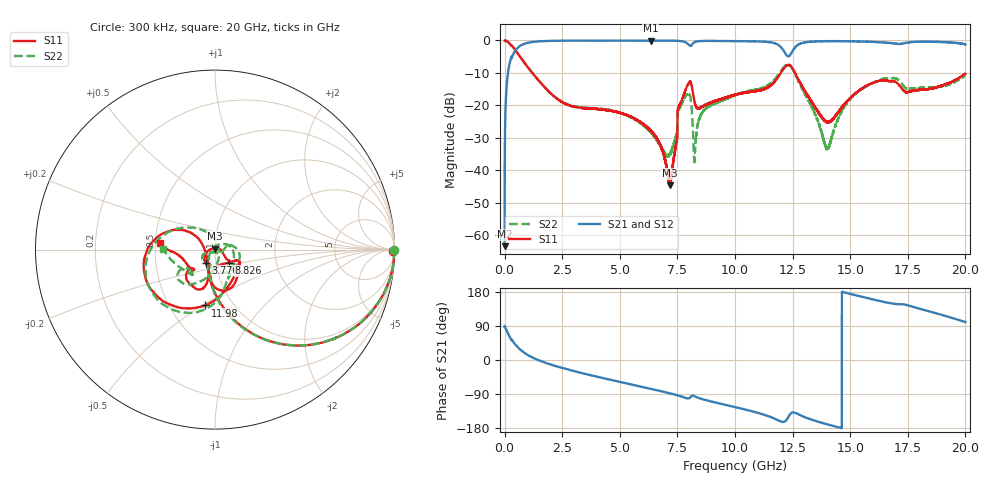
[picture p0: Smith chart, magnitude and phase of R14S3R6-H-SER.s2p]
!{R14S3R6}
!Johanson Technology Inc.
!www.johansontechnology.com
!Test Board Conditions:
!Substrate Type  RO4350B
!Substrate Thickness  20 mil
!Substrate Dk  3.66
!TL Type: GCPW
!TL Trace Width  36 mil
!TL Gap  12 mil
!Electrode orientation  Horizontal
!DUT TOPOLOGY	SERIES
!Mounting Pad LxW  26x36 mil
! Created Wed Nov 25 17:33:21 2020
! 2 Port Network Data from SP1.SP block
! freq  magS11  angS11  magS21  angS21  magS12  angS12  magS22  angS22
# khz S ma R 50
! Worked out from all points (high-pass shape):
!   20001 points, 300 kHz to 20 GHz, reference 50 ohm
!   highest |S21| = -0.05 dB at 6.349 GHz (marker M1); lowest = -63.4 dB at 300 kHz (marker M2)
!   |S21| within 3 dB of the highest: 471 MHz to 12.1 GHz (11.63 GHz wide, 185 % of centre); 12.51 GHz to end of sweep
!   lowest |S11| = -44.6 dB at 7.16 GHz (marker M3), VSWR 1.01, Z = 50 + j0.585 ohm
!   |S11| at or under -10 dB: 1.2 GHz to 11.98 GHz (10.78 GHz wide, 164 % of centre); 12.61 GHz to end of sweep
!   |S22| runs from -37.6 to 0.0 dB; largest |S21 - S12| = 0.018
!   S11 on the Smith chart (normalised r, x): 300 kHz: open; 3.776 GHz: 0.89, -0.13; 8.826 GHz: 1.15, -0.17; 11.98 GHz: 0.74, -0.51; 20 GHz: 0.53, +0.04
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300  0.9935 -0.3  0.0006738 86.8  0.0006502 88.8  0.9982 -0.2
118300  0.965 -16.3  0.259 73.5  0.2597 73.5  0.9648 -16.3
370300  0.7873 -41.2  0.611 48.5  0.6122 48.5  0.7874 -41.2
1252300  0.2998 -84.2  0.9516 5.3  0.9514 5.3  0.3014 -84.9
3334300  0.09133 -121.0  0.9923 -34.2  0.9929 -34.2  0.09262 -125.7
3776300  0.08892 -125.7  0.9919 -40.7  0.9922 -40.7  0.09011 -134.0
6349300  0.04073 -169.2  0.9945 -76.1  0.993 -76.1  0.03808 -156.4
6667300  0.02803 -179.8  0.9932 -80.6  0.9931 -80.6  0.02671 -146.9
7160300  0.005862 92.5  0.9919 -87.7  0.9918 -87.7  0.01722 -83.6
7600300  0.1015 -38.3  0.9797 -94.9  0.9801 -94.9  0.0919 15.3
7946300  0.2054 -54.5  0.8889 -101.4  0.8886 -101.3  0.146 -30.9
8263300  0.1058 -91.7  0.9498 -96.3  0.95 -96.2  0.01989 82.6
8826300  0.1056 -43.9  0.9831 -107.2  0.984 -107.3  0.09488 3.1
1.00003e7  0.1454 -25.0  0.9776 -124.3  0.9784 -124.3  0.143 -48.6
1.19833e7  0.3163 -100.0  0.7967 -162.3  0.8006 -162.2  0.3355 -98.9
1.24153e7  0.4048 -169.2  0.6131 -141.1  0.6169 -141.5  0.4006 -165.1
1.33343e7  0.1122 145.7  0.9589 -157.6  0.9576 -157.6  0.09387 110.6
1.40203e7  0.05458 -165.1  0.9767 -170.0  0.9757 -170.0  0.0219 4.5
1.50073e7  0.1305 -104.8  0.9708 174.4  0.9725 174.2  0.1265 -97.6
1.66673e7  0.2357 -121.9  0.9189 150.8  0.9108 150.8  0.2614 -136.2
1.74853e7  0.1602 -136.8  0.928 144.5  0.9285 144.3  0.1802 -141.8
2e7  0.3076 173.4  0.8676 100.2  0.8689 100.3  0.2887 179.0
